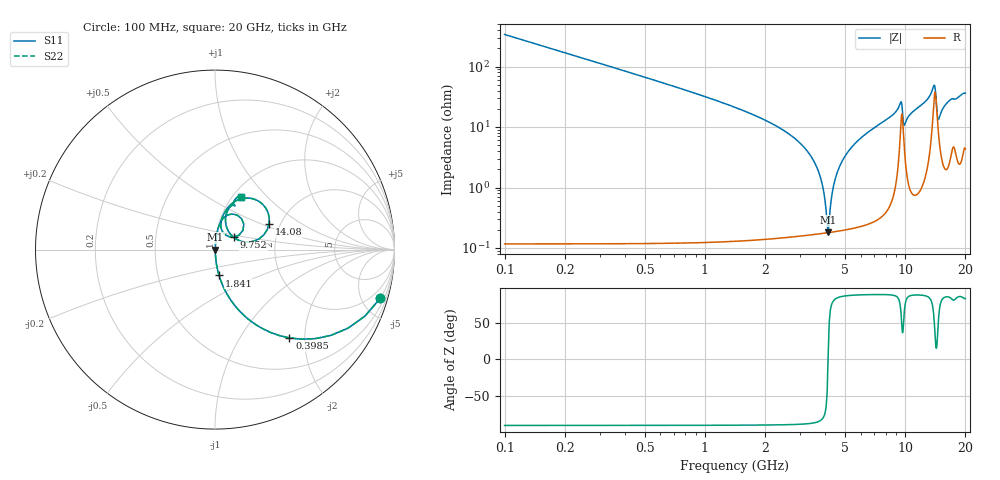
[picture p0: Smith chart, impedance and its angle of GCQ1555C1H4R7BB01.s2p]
!Murata Part Number: GCQ1555C1H4R7BB01
!These Parameters are Measured in Series Mode Connection
!Data Generated on Mar 13, 2026
!  o--ll--o
!Port1  Port2
!  o------o
!Operation Temp=25[degC], DC Bias Voltage=0[V]
!Freq. Start=100[MHz] Stop=20[GHz] 401[Steps]
# Hz S RI R 50
!Freq.(Hz) S11(Real) S11(Imag) S21(Real) S21(Imag) S12(Real) S12(Imag) S22(Real) S22(Imag)
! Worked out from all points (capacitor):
!   401 points, 100 MHz to 20 GHz, reference 50 ohm
!   read as one part in series: C = 4.7 pF near 199.5 MHz
!   lowest |Z| = 181 mohm at 4.13 GHz (marker M1)
!   series resonance near 4.124 GHz, so ESL is about 320 pH
!   S11 on the Smith chart (normalised r, x): 100 MHz: 1.00, -6.77; 398.5 MHz: 1.00, -1.68; 1.841 GHz: 1.00, -0.30; 9.752 GHz: 1.22, +0.17; 14.08 GHz: 1.75, +0.56; 20 GHz: 1.09, +0.72
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1e8  0.9196 -0.2717  0.0804 0.2717  0.0804 0.2717  0.9196 -0.2717
3.985e8  0.4149 -0.492  0.5851 0.492  0.5851 0.492  0.4149 -0.492
8.4625e8  0.129 -0.3336  0.871 0.3336  0.871 0.3336  0.129 -0.3336
1.84125e9  0.0226 -0.144  0.9774 0.144  0.9774 0.144  0.0226 -0.144
3.43325e9  0.00258 -0.0304  0.9974 0.0304  0.9974 0.0304  0.00258 -0.0304
3.7815e9  0.00193 -0.0144  0.9981 0.0144  0.9981 0.0144  0.00193 -0.0144
4.03025e9  0.00179 -0.00382  0.9982 0.00382  0.9982 0.00382  0.00179 -0.00382
4.12975e9  0.00179 0.000225  0.9982 -0.000225  0.9982 -0.000225  0.00179 0.000225
4.478e9  0.00205 0.0137  0.9979 -0.0137  0.9979 -0.0137  0.00205 0.0137
4.876e9  0.00274 0.0281  0.9973 -0.0281  0.9973 -0.0281  0.00274 0.0281
5.62225e9  0.00496 0.0529  0.995 -0.0529  0.995 -0.0529  0.00496 0.0529
6.7665e9  0.0104 0.0882  0.9896 -0.0882  0.9896 -0.0882  0.0104 0.0882
9.453e9  0.1084 0.1964  0.8916 -0.1964  0.8916 -0.1964  0.1084 0.1964
9.7515e9  0.106 0.0698  0.894 -0.0698  0.894 -0.0698  0.106 0.0698
9.90075e9  0.0532 0.0866  0.9468 -0.0866  0.9468 -0.0866  0.0532 0.0866
1.005e10  0.0372 0.1103  0.9628 -0.1103  0.9628 -0.1103  0.0372 0.1103
1.338325e10  0.1374 0.2806  0.8626 -0.2806  0.8626 -0.2806  0.1374 0.2806
1.378125e10  0.2324 0.2754  0.7676 -0.2754  0.7676 -0.2754  0.2324 0.2754
1.407975e10  0.3012 0.143  0.6988 -0.143  0.6988 -0.143  0.3012 0.143
1.4627e10  0.0895 0.0821  0.9105 -0.0821  0.9105 -0.0821  0.0895 0.0821
1.67165e10  0.0918 0.2443  0.9082 -0.2443  0.9082 -0.2443  0.0918 0.2443
2e10  0.1437 0.2955  0.8563 -0.2955  0.8563 -0.2955  0.1437 0.2955
